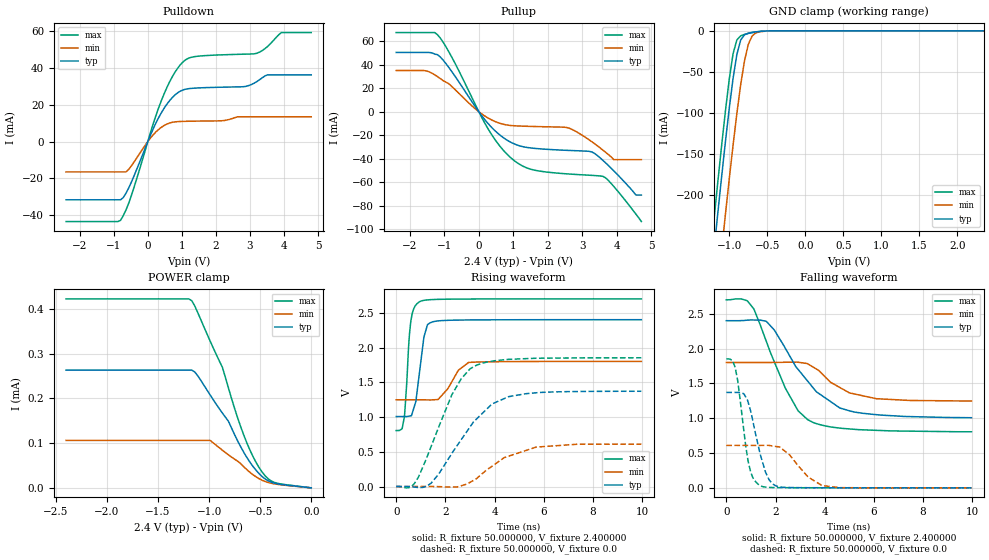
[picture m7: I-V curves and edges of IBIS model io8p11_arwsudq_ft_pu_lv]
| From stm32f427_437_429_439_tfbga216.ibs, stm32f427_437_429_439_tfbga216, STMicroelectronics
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|   Model io8p11_arwsudq_ft_pu_lv
[Model]  io8p11_arwsudq_ft_pu_lv
Model_type I/O
Polarity   Non-Inverting
Enable   Active-Low
Vinl =   0.720000V
Vinh =   1.680000V
Vmeas =  1.200000V
Cref =   30.000000pF
Rref =   100.000000M
Vref =   0.0V
C_comp   2.828100pF   2.774600pF   2.917100pF
[Temperature Range]   25.000000   0.125000k   -40.000000
[Pullup Reference]   2.400000V   1.800000V   2.700000V
[Pulldown Reference]   0.0V   0.0V   0.0V
[POWER Clamp Reference]   2.400000V   1.800000V   2.700000V
[GND Clamp Reference]   0.0V   0.0V   0.0V
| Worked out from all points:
|   slope of the pulldown table from 0 to 0.36 V, typ, clamps not added: 25 ohm
|   slope of the pullup table from 0 to 0.36 V, typ, clamps not added: 27.7 ohm
|   GND clamp passes 1 mA (typ) near -0.62 V on its own axis
|   rising waveform, R_fixture 50.000000, V_fixture 2.400000: 20-80 % time 295ps typ, 615ps min, 205ps max; typ from 1.01 V to 2.4 V
|   rising waveform, R_fixture 50.000000, V_fixture 0.0: 20-80 % time 1.73ns typ, 1.72ns min, 1.34ns max; typ from 0.001 V to 1.37 V
|   falling waveform, R_fixture 50.000000, V_fixture 2.400000: 20-80 % time 1.85ns typ, 1.34ns min, 1.4ns max; typ from 2.4 V to 1.01 V
|   falling waveform, R_fixture 50.000000, V_fixture 0.0: 20-80 % time 558ps typ, 950ps min, 411ps max; typ from 1.37 V to 0.001 V
[Pulldown]
|Voltage   I(typ)   I(min)   I(max)
-2.4V     -31.67mA   -16.51mA   -43.52mA
-800mV    -31.67mA   -16.51mA   -42.87mA
-480mV    -21.98mA   -13.17mA   -29.21mA
80mV      3.63mA     1.966mA    5.012mA
480mV     18.16mA    8.738mA    26.02mA
800mV     25.38mA    10.72mA    37.77mA
1.12V     28.53mA    11.02mA    44.6mA
2.8V      29.84mA    13.46mA    47.53mA
3.2V      32.6mA     13.46mA    48.03mA
3.52V     36.31mA    13.46mA    51.75mA
3.92V     36.31mA    13.46mA    59.29mA
4.8V      36.31mA    13.46mA    59.29mA
[Pullup]
|Voltage   I(typ)   I(min)   I(max)
-2.4V     50.44mA    35.08mA    67.37mA
-1.52V    50.44mA    34.74mA    67.37mA
-1.2V     48.54mA    29.87mA    65.51mA
320mV     -11.75mA   -6.207mA   -17.08mA
1.04V     -27.53mA   -11.97mA   -41.91mA
1.6V      -31.13mA   -12.57mA   -49.63mA
2.56V     -32.88mA   -13.48mA   -52.9mA
3.28V     -34.19mA   -25.52mA   -54.17mA
3.6V      -41.32mA   -32.62mA   -54.98mA
3.92V     -50.33mA   -40.8mA    -63.65mA
4.56V     -70.9mA    -40.8mA    -87.11mA
4.72V     -70.9mA    -40.8mA    -93.5mA
[GND_clamp]
|Voltage   I(typ)   I(min)   I(max)
-2.4V     -1.425A    -1.508A    -1.394A
-1.25V    -311.8mA   -402mA     -274.5mA
-1.2V     -266mA     -356.2mA   -228.4mA
-1.15V    -220.9mA   -310.9mA   -183.1mA
-1.1V     -176.9mA   -266.3mA   -139mA
-1.05V    -134.3mA   -222.6mA   -97.01mA
-950mV    -57.81mA   -139.1mA   -27.86mA
-900mV    -28.73mA   -100.5mA   -11.04mA
-850mV    -11.29mA   -65.69mA   -6.054mA
-750mV    -2.852mA   -16.6mA    -3.179mA
-600mV    -750uA     -1.167mA   -738.5uA
2.35V     0A         0A         0A
[POWER_clamp]
|Voltage   I(typ)   I(min)   I(max)
-2.4V     263.2uA    106uA      422.4uA
-1.17V    263.2uA    106uA      418.5uA
-1.11V    250.1uA    106uA      391.1uA
-990mV    207.7uA    106uA      328.2uA
-870mV    167.2uA    84.17uA    269.6uA
-810mV    148.5uA    73.71uA    222.7uA
-660mV    79.21uA    47.09uA    117.6uA
-570mV    47.82uA    29.3uA     69.9uA
-510mV    31.66uA    20.4uA     45.18uA
-420mV    15.55uA    11.87uA    19.89uA
-360mV    10.34uA    8.845uA    12.09uA
0V        0A         0A         0A
[Ramp]
| variable   typ   min   max
dV/dt_r  0.82165/1.72943n   0.36425/1.70946n   1.11088/1.33754n
dV/dt_f  0.83172/1.84083n   0.33198/1.35349n   1.13512/1.39505n
R_load = 50.000000
[Rising Waveform]
R_fixture= 50.000000
V_fixture= 2.400000
V_fixture_min= 1.800000
V_fixture_max= 2.700000
|time   V(typ)   V(min)   V(max)
0s        1.007V     1.247V     805.7mV
240.2ps   1.007V     1.247V     830.8mV
320.3ps   1.007V     1.247V     980.6mV
580.6ps   1.017V     1.247V     2.337V
800.8ps   1.227V     1.247V     2.611V
940.9ps   1.624V     1.247V     2.656V
1.141ns   2.168V     1.247V     2.679V
1.502ns   2.371V     1.248V     2.69V
2.943ns   2.396V     1.785V     2.697V
9.97ns    2.4V       1.8V       2.699V
[Rising Waveform]
R_fixture= 50.000000
V_fixture= 0.0
V_fixture_min= 0.0
V_fixture_max= 0.0
|time   V(typ)   V(min)   V(max)
0s        1.052mV    906.2uV    1.473mV
740.7ps   -6.701mV   896.6uV    44.24mV
1.421ns   49.55mV    994.2uV    578.1mV
2.282ns   487.7mV    -5.979mV   1.333V
2.643ns   674mV      11.76mV    1.55V
3.203ns   950.2mV    101.3mV    1.734V
3.904ns   1.189V     294.6mV    1.804V
4.384ns   1.264V     414.9mV    1.824V
5.686ns   1.349V     567.2mV    1.845V
9.97ns    1.371V     610.1mV    1.852V
[Falling Waveform]
R_fixture= 50.000000
V_fixture= 2.400000
V_fixture_min= 1.800000
V_fixture_max= 2.700000
|time   V(typ)   V(min)   V(max)
0s        2.4V       1.8V       2.699V
840.8ps   2.407V     1.8V       2.687V
1.121ns   2.41V      1.8V       2.567V
1.622ns   2.392V     1.8V       2.107V
2.402ns   2.002V     1.804V     1.43V
2.923ns   1.699V     1.804V     1.105V
3.323ns   1.526V     1.778V     976.8mV
4.605ns   1.15V      1.443V     858.9mV
5.085ns   1.099V     1.358V     844.3mV
9.97ns    1.007V     1.247V     805.7mV
[Falling Waveform]
R_fixture= 50.000000
V_fixture= 0.0
V_fixture_min= 0.0
V_fixture_max= 0.0
|time   V(typ)   V(min)   V(max)
0s        1.371V     610.1mV    1.852V
360.4ps   1.371V     610.2mV    1.728V
460.5ps   1.37V      610.1mV    1.543V
860.9ps   1.258V     610mV      439.8mV
1.061ns   991.2mV    609.8mV    160.5mV
1.381ns   478mV      610.1mV    31.9mV
1.742ns   115.5mV    609.1mV    7.813mV
2.182ns   13.89mV    582.9mV    4.208mV
3.904ns   2.275mV    33.59mV    2.192mV
9.97ns    1.052mV    906.2uV    1.473mV
